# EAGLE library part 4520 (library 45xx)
Dual binary up COUNTER
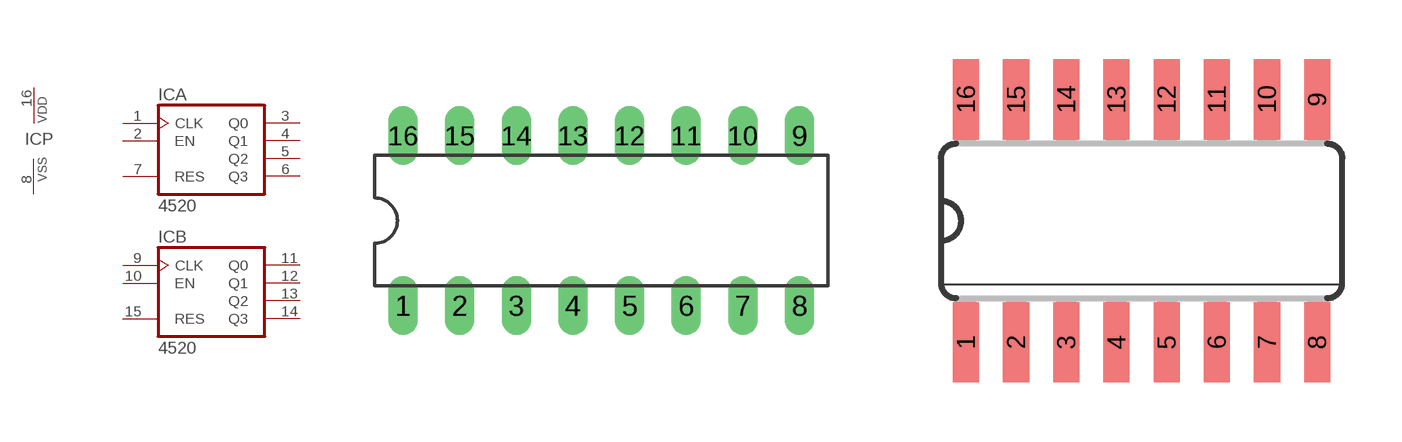
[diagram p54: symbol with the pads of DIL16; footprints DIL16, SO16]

Designator prefix IC; gates A=4518 B=4518 P=PWRN

## 4520N  [DIL16]
1  A:CLK  in
2  A:EN  in
3  A:Q0  out
4  A:Q1  out
5  A:Q2  out
6  A:Q3  out
7  A:RES  in
8  P:VSS  pwr
9  B:CLK  in
10  B:EN  in
11  B:Q0  out
12  B:Q1  out
13  B:Q2  out
14  B:Q3  out
15  B:RES  in
16  P:VDD  pwr

## 4520D  [SO16]
Pads as for DIL16

## Footprint DIL16 (pad centres in mm)
Dual In Line Package
drill 0.813 long: 1 -8.89,-3.81; 2 -6.35,-3.81; 3 -3.81,-3.81; 4 -1.27,-3.81; 5 1.27,-3.81; 6 3.81,-3.81; 7 6.35,-3.81; 8 8.89,-3.81; 9 8.89,3.81; 10 6.35,3.81; 11 3.81,3.81; 12 1.27,3.81; 13 -1.27,3.81; 14 -3.81,3.81; 15 -6.35,3.81; 16 -8.89,3.81

## Footprint SO16 (pad centres in mm)
Small Outline package 150 mil
smd 0.66 x 2.032: 1 -4.445,-3.073; 2 -3.175,-3.073; 3 -1.905,-3.073; 4 -0.635,-3.073; 5 0.635,-3.073; 6 1.905,-3.073; 7 3.175,-3.073; 8 4.445,-3.073; 9 4.445,3.073; 10 3.175,3.073; 11 1.905,3.073; 12 0.635,3.073; 13 -0.635,3.073; 14 -1.905,3.073; 15 -3.175,3.073; 16 -4.445,3.073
